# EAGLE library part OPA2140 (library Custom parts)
Dual Operational Amplifier Low Power, Single-Supply, Rail-To-Rail Operational Amplifier Source: http://focus.ti.com/lit/ds/symlink/opa2345.pdf http://focus.ti.com .. opa241.pdf http://focus.ti.com/lit/ds/symlink/opa2134.pdf
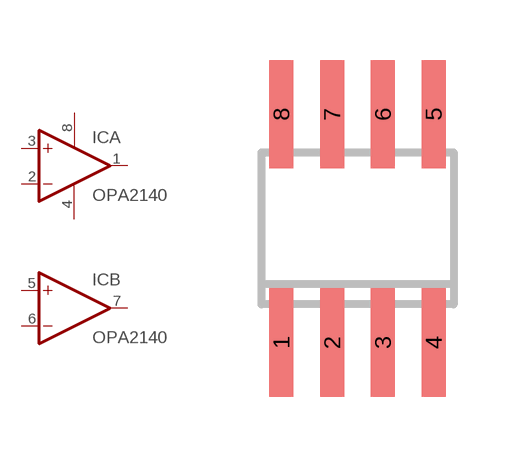
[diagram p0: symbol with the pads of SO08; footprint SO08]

Designator prefix IC; gates A=OPAMP+- B=OPAMP

## OPA2140  [SO08]
1  A:OUT  out
2  A:-IN  in
3  A:+IN  in
4  A:V-  pwr
5  B:+IN  in
6  B:-IN  in
7  B:OUT  out
8  A:V+  pwr

## Footprint SO08 (pad centres in mm)
Small Outline Package 8 NS Package M08A
smd 0.6 x 2.708: 1 -1.905,-2.854; 2 -0.635,-2.854; 3 0.635,-2.854; 4 1.905,-2.854; 5 1.905,2.854; 6 0.635,2.854; 7 -0.635,2.854; 8 -1.905,2.854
